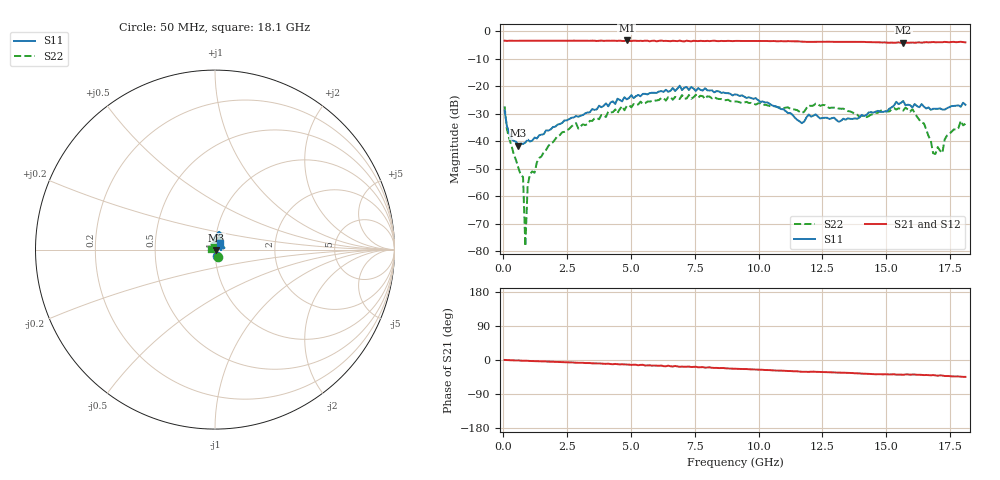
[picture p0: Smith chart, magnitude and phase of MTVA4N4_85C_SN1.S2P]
! Network Analyzer HP8720D.06.14 Serial No. US36140669
! 28 Jun 2005  10:25:00
! Frequency  S11  S21  S12  S22
# HZ  S  DB R 50
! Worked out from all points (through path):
!   201 points, 50 MHz to 18.1 GHz, reference 50 ohm
!   highest |S21| = -3.35 dB at 4.833 GHz (marker M1); lowest = -4.2 dB at 15.66 GHz (marker M2)
!   group delay of S21, straight-line fit = 6.9 ps
!   lowest |S11| = -41.6 dB at 591.5 MHz (marker M3), VSWR 1.02, Z = 50.8 - j0.226 ohm
!   |S11| at or under -10 dB: start of sweep to end of sweep
!   |S22| runs from -78.2 to -23.1 dB; largest |S21 - S12| = 0.019
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5e7  -28.82 -67.9  -3.42 0.2  -3.43 0.2  -27.32 -63.5
1.4025e8  -34.51 -57.2  -3.50 -0.1  -3.48 -0.2  -35.68 -74.2
5.915e8  -41.60 -15.5  -3.44 -1.2  -3.47 -1.2  -49.79 -45.2
7.72e8  -41.00 0.8  -3.46 -1.9  -3.44 -1.7  -53.05 -24.8
8.6225e8  -40.52 1.2  -3.45 -1.9  -3.47 -1.9  -78.19 49.5
9.525e8  -39.39 4.4  -3.47 -2.1  -3.45 -2.2  -56.22 29.3
1.04275e9  -40.10 13.7  -3.44 -2.6  -3.44 -2.4  -51.96 35.4
2.12575e9  -33.96 31.7  -3.44 -5.2  -3.44 -5.2  -38.12 79.6
3.1185e9  -30.45 47.4  -3.44 -7.4  -3.46 -7.7  -33.85 96.3
4.83325e9  -24.77 65.8  -3.35 -11.8  -3.43 -12.3  -27.22 80.3
6.09675e9  -21.91 68.2  -3.48 -15.2  -3.42 -15.2  -25.00 76.5
9.075e9  -22.95 89.2  -3.53 -22.8  -3.51 -22.9  -25.51 58.6
1.169225e10  -33.44 111.3  -3.77 -31.1  -3.77 -31.0  -29.74 78.0
1.21435e10  -30.73 96.8  -3.89 -30.7  -3.85 -31.0  -27.05 84.6
1.313625e10  -32.92 58.3  -3.89 -33.2  -3.85 -33.5  -28.11 87.4
1.512175e10  -28.18 14.0  -4.17 -38.2  -4.09 -38.0  -29.17 121.5
1.566325e10  -25.36 10.5  -4.21 -39.1  -4.16 -38.2  -28.86 100.4
1.64755e10  -27.44 26.9  -4.06 -39.8  -4.19 -39.0  -33.54 64.5
1.692675e10  -28.19 39.6  -4.00 -40.6  -3.90 -40.6  -44.66 89.5
1.71975e10  -28.50 38.3  -3.99 -41.0  -3.93 -40.2  -44.29 149.4
1.79195e10  -27.50 56.9  -3.83 -44.0  -3.73 -43.6  -32.60 164.1
1.81e10  -26.76 52.3  -4.05 -44.5  -4.06 -45.4  -33.69 172.4
